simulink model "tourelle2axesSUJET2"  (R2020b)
settings: Solver=VariableStepAuto  StartTime=0.0  StopTime=0.2  RelTol=1e-3  AbsTol=1e-3
libraries: nesl_utility x7, fl_lib x6, ee_lib x3, batteryecm_lib x1, sdl_lib x1

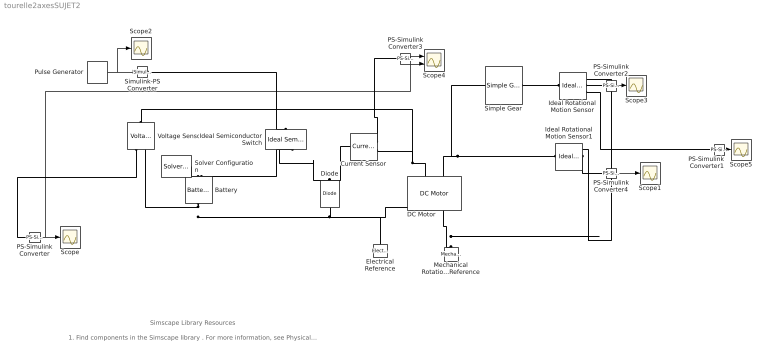
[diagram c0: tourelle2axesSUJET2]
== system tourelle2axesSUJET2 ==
  note: 1. Find components in the Simscape library . For more information, see Physical Modeling - Blocks . 2. Connect the components to form a physical network. For more information, see Essential Steps for Constructing a Physical Model . 3. Explore simulation results using sscexplore
  note: Simscape Library Resources
  Battery : batteryecm_lib/Battery  Vnom=3.93 V  prm_dir=simscape.enum.battery.prm_dir.disabled  R1_dis=2 Ohm  R1_ch=2 Ohm  R1=0.06 Ohm  prm_AH=2  AH=0.750 hr*A  V1=3.8 V  AH1=0.3 hr*A  prm_R2=simscape.enum.battery.prm_R2.enabled  R2=inf Ohm  Tmeas=298.15 K  charge_measurement_port=simscape.enum.battery.enable.no  prm_dyn=1  Rp1=0.005 Ohm  tau1=30 s  Rp2=0.005 Ohm  tau2=30 s  Rp3=0.005 Ohm  tau3=30 s  Rp4=0.005 Ohm  tau4=30 s  Rp5=0.005 Ohm  tau5=30 s  prm_fade=1  N_fade=100  AH_fade=45 hr*A  R1_fade=2.02 Ohm  R1_ch_fade=2.02 Ohm  V1_fade=10.35 V  prm_age=simscape.enum.battery.prm_age.disabled  prm_age_OCV=simscape.enum.battery.prm_age_OCV.OCV  OCV_age=0.9  SOC_age=60  Tmeas_age=298.15 K  delta_time_age_vec=[0] d  temperature_age_vec=[273] K  OCV_scaling_age=2.2134e6  OCV_offset_age=1.632e6  temp_exp_age=0.515833569 V  t_exp_age=0.75  Vnom_T2=12 V  R1_T2=2.2 Ohm  R1_T2_dis=2.2 Ohm  R1_T2_ch=2.2 Ohm  V1_T2=11.4 V  R2_T2=2200 Ohm  Rp1_T2=0.005 Ohm  tau1_T2=30 s  Rp2_T2=0.005 Ohm  tau2_T2=30 s  Rp3_T2=0.005 Ohm  tau3_T2=30 s  Rp4_T2=0.005 Ohm  tau4_T2=30 s  Rp5_T2=0.005 Ohm  tau5_T2=30 s  Tmeas2=273.15 K  thermal_port=simscape.enum.thermaleffects.omit  thermal_mass=30000 J/K  i_specify=off  i_priority=None  i=0 A  i_nominal_specify=off  i_nominal_value=1  i_nominal_unit=A  v_specify=off  v_priority=None  v=0 V  v_nominal_specify=off  v_nominal_value=1  v_nominal_unit=V  charge_specify=off  charge_priority=High  charge=50 hr*A  charge_nominal_specify=off  charge_nominal_value=1  charge_nominal_unit=hr*A  num_cycles_specify=off  num_cycles_priority=High  num_cycles=0  num_cycles_nominal_specify=off  num_cycles_nominal_value=1  num_cycles_nominal_unit=1  temperature_specify=off  temperature_priority=High  temperature=298.15 K  temperature_nominal_specify=off  temperature_nominal_value=1  temperature_nominal_unit=K
  Current Sensor : fl_lib/Electrical/Electrical Sensors/Current Sensor
  DC Motor : ee_lib/Electromechanical/Brushed Motors/DC Motor  field_option=ee.enum.field_option.pm  Rf=100 Ohm  Lf=1 H  Laf=0.15 H  If0=0 A  parameterization=1  Ra=79 Ohm  La=3 mH  emf_or_torque=1  Kv=0.0145 V/(rad/s)  Ki=6.876e-4 N*m/A  T_stall=0.24e-3 N*m  w_max=19100 rpm  w_rated=15000 rpm  P_rated=0.08 W  V_rated=1.5 V  lam_param=1  i_noload=0 A  V_i_noload=1.5 V  J=1 g*cm^2  lam=0 N*m/(rad/s)  speed0=0 rpm  enable_fault_armature=simscape.enum.onoff.off  rev_faulted=1 / 3  G_faulted_armature=1e-5 S  fault_trigger_armature=ee.enum.faults.faultTrigger.temporal  t_fault_armature=1 s  max_permissible_current_armature=inf A  t_fail_on_current_armature=1 s  enable_fault_field=simscape.enum.onoff.off  G_faulted_field=1e-5 S  fault_trigger_field=ee.enum.faults.faultTrigger.temporal  t_fault_field=1 s  max_permissible_current_field=inf A  t_fail_on_current_field=1 s  fault_action=simscape.enum.assert.action.none  alpha=3.93e-3 1/K  Tmeas=25 degC  thermal_mass=100 J/K  initial_temperature=25 degC
  Diode : ee_lib/Semiconductors & Converters/Diode  ModelType=ee.enum.diode.modelType.pwl  TableType=ee.enum.diode.tableType.IfMat  IfMat=[.07, .12, .19, 1.75, 4.24, 7.32, 11.2; .16, .3, .72, 2.14, 5.02, 8.35, 13.12] A  VfMat=[.9, 1.15, 1.25, 1.5, 1.75, 2.17, 2.6, 2.85; .58, .68, .75, 1.1, 1.38, 1.77, 2.27, 2.7] V  TjVec=[25, 125] degC  VfVec=[.5, .7, .9, 1.3, 1.7, 2.1, 2.5] V  IfVec=[.1, .2, .5, 1, 2, 4, 7, 10] A  IrMat=[1e-06, 2e-06, 5e-06, 1e-05, 2.5e-05, 5e-05, .0001; 2e-06, 5e-06, 1e-05, 4e-05, 8e-05, .0002, .0005] A  VrMat=[10, 100, 200, 250, 300, 325, 350; 10, 70, 160, 220, 270, 300, 320] V  VrVec=[10, 20, 40, 50, 70, 80, 100] V  IrVec=[1e-06, 2e-06, 5e-06, 1e-05, 2e-05, 5e-05, .0001] A  Vf=0.6 V  Ron=0.3 Ohm  Goff=1e-8 S  prmExp=ee.enum.diode.expParam.useTwo  I12=[.0137, .545] A  V12=[.6, .7] V  RS=0 Ohm  Tmeas=25 degC  IS=1e-12 A  ec=1  I1=0.0137 A  V1=0.6 V  N_series=1  N_parallel=1  ZenerEnable=false  Rz=0.3 Ohm  BV=inf V  C_param=ee.enum.diode.capParam.fixed  CJ=5 pF  CJ0=5 pF  Vvec=[.1, 10, 100] V  Cvec=[3.5, 1, .4] pF  VJ=1 V  Mgrad=0.5  FC=0.5  Q_param=ee.enum.diode.recoveryParam.off  iRM=-7.15 A  iF=4 A  didt=-750 A/us  trr_factor=3  trr=115 ns  Qrr=1500 s*uA  Vr=-600 V  Ls=150 nH  Erec=0.03 J  TT=50 ns  tau=100 ns  T_param=ee.enum.diode.temperatureParam.off  Tdevice=25 degC  I1_T2=0.245 A  V1_T2=0.5 V  IS_T2=1.25e-7 A  Tmeas2=125 degC  XTI_param=ee.enum.diode.xtiParam.pn  XTI=3  EG_param=ee.enum.diode.egapParam.material_si  EG=1.11 eV  dBVdT=0 V/K  enable_faults=simscape.enum.onoff.off  fault_action=simscape.enum.assert.action.none  fault_types=ee.enum.diode.faults.open  tau_fault=1e-3 s  IfMat_faulted=[.07, .12, .19, 1.75, 4.24, 7.32, 11.2; .16, .3, .72, 2.14, 4.02, 6.35, 9.12] A  VfMat_faulted=[.9, 1.15, 1.25, 1.5, 1.75, 2.17, 2.6, 2.85; .58, .68, .75, 1.1, 1.38, 1.77, 2.27, 2.7] V  VfVec_faulted=[.5, .7, .9, 1.3, 1.7, 2.1, 2.5] V  IfVec_faulted=[.1, .2, .5, 1, 2, 4, 7, 10] A  IrMat_faulted=[1e-06, 2e-06, 5e-06, 1e-05, 2.5e-05, 5e-05, .0001; 2e-06, 5e-06, 1e-05, 4e-05, 8e-05, .0002, .0005] A  VrMat_faulted=[1, 10, 20, 25, 30, 32.5, 35; 1, 5, 10, 20, 25, 30, 32] V  VrVec_faulted=[1, 2, 4, 5, 7, 8, 10] V  IrVec_faulted=[1e-06, 2e-06, 5e-06, 1e-05, 2e-05, 5e-05, .0001] A  Ropen_faulted=1000 Ohm  Gshort_faulted=1000 1/Ohm  Vf_faulted=0.6 V  Ron_faulted=0.3 Ohm  Goff_faulted=1e-8 S  I12_faulted=[.0137, .545] A  V12_faulted=[.6, .7] V  IS_faulted=1e-12 A  ec_faulted=1  I1_faulted=0.0137 A  V1_faulted=0.6 V  RS_faulted=0 Ohm  Rz_faulted=0.3 Ohm  BV_faulted=inf V  Cscale_faulted=100  fault_trigger=ee.enum.faults.faultTrigger.temporal  t_fault=inf s  max_permissible_voltage=inf V  n_fail_on_voltage=1  max_permissible_current=inf A  t_fail_on_current=1 s  max_permissible_dVdt=inf V/s  enable_fault_input=simscape.enum.onoff.off  i_specify=off  i_priority=None  i=0 A  i_nominal_specify=off  i_nominal_value=1  i_nominal_unit=A  v_specify=off  v_priority=None  v=0 V  v_nominal_specify=off  v_nominal_value=1  v_nominal_unit=V  v_capacitor_specify=off  v_capacitor_priority=None  v_capacitor=0 V  v_capacitor_nominal_specify=off  v_capacitor_nominal_value=1  v_capacitor_nominal_unit=V  Qj_specify=off  Qj_priority=High  Qj=0 C  Qj_nominal_specify=off  Qj_nominal_value=1  Qj_nominal_unit=C  faulted_specify=off  faulted_priority=None  faulted=0  faulted_nominal_specify=off  faulted_nominal_value=1  faulted_nominal_unit=1  i_diode_specify=off  i_diode_priority=None  i_diode=0 A  i_diode_nominal_specify=off  i_diode_nominal_value=1  i_diode_nominal_unit=A  v_diode_specify=off  v_diode_priority=None  v_diode=0 V  v_diode_nominal_specify=off  v_diode_nominal_value=1  v_diode_nominal_unit=V  i_capacitor_specify=off  i_capacitor_priority=None  i_capacitor=0 A  i_capacitor_nominal_specify=off  i_capacitor_nominal_value=1  i_capacitor_nominal_unit=A  power_dissipated_specify=off  power_dissipated_priority=None  power_dissipated=0 W  power_dissipated_nominal_specify=off  power_dissipated_nominal_value=1  power_dissipated_nominal_unit=W  fidelity_level=ee.enum.diode.fidelity.includeChargeDyn  rec_loss_model=ee.enum.diode.reverseRecoveryModel.fixed  ErecVal=0 J  scaleWithIandV=true  ErecMat=zeros(2, 3) J  TjrecVec=[298.15, 398.15] K  IfrecVec=[.1, 1, 10] A  IrecVal=10 A  VrecVal=10 V  tFilter=1 / 1000 / 100 s  max_permissible_temperature=inf K  t_fail_on_temperature=1 s  thermal_network_parameterization=ee.enum.thermalNetworkTopology.cauer  Rth=[0, 10] K/W  Rth_Cauer=[1, 3, 10] K/W  Rth_Foster=[4, 6] K/W  thermal_mass_parameterization=ee.enum.thermalNetwork.timeconstant  thermal_mass=[0, 1] J/K  thermal_mass_Cauer=[.1, .3, 1] J/K  thermal_mass_Foster=[1.5, 3] J/K  thermal_time_constant=[0, 10] s  thermal_time_constant_Cauer=[1, 3, 10] s  thermal_time_constant_Foster=[6, 18] s  thermal_mass_initial_temperatures=[25, 25] degC  thermal_mass_initial_temperatures_Cauer=[25, 25, 25] degC  junction_thermal_mass=0.01 J/K  Tvec_initial_Foster=[25, 25, 25, 25] degC  no_thermal_network=0  junction_temperature_specify=off  junction_temperature_priority=None  junction_temperature=25 degC  junction_temperature_nominal_specify=off  junction_temperature_nominal_value=1  junction_temperature_nominal_unit=degC
  Electrical Reference : fl_lib/Electrical/Electrical Elements/Electrical Reference
  Ideal Rotational Motion Sensor : fl_lib/Mechanical/Mechanical Sensors/Ideal Rotational Motion Sensor  reference=foundation.enum.MeasurementReference.difference  acceleration_port=false  velocity_port=true  position_port=true  wrap_angle=false  offset=0 rad
  Ideal Rotational Motion Sensor1 : fl_lib/Mechanical/Mechanical Sensors/Ideal Rotational Motion Sensor  reference=foundation.enum.MeasurementReference.difference  acceleration_port=false  velocity_port=true  position_port=true  wrap_angle=false  offset=0 rad
  Ideal Semiconductor Switch : ee_lib/Semiconductors & Converters/Ideal Semiconductor Switch  port_option=ee.enum.controlport.ps  Ron=0.001 Ohm  Goff=1e-6 1/Ohm  Vth=0.5 V  diode_param=1  diode_Vf=0.8 V  diode_Ron=0.001 Ohm  diode_Goff=1e-5 1/Ohm  diode_C=50e-9 F  diode_iRM=-235 A  diode_iF=300 A  diode_idot=-50 A/us  diode_trr_param=1  diode_trr_factor=3  diode_trr=15 us  diode_Qrr=1500 s*uA
  Mechanical Rotational Reference : fl_lib/Mechanical/Rotational Elements/Mechanical Rotational Reference
  PS-Simulink Converter : nesl_utility/PS-Simulink Converter  PhysicalDomain=network_engine_domain  SubClassName=ps_output  LeftPortType=input  RightPortType=output  PseudoPeriodic=off  Frequencies=[]  VectorFormat=1-D array  Unit=V  AffineConversion=off
  PS-Simulink Converter1 : nesl_utility/PS-Simulink Converter  PhysicalDomain=network_engine_domain  SubClassName=ps_output  LeftPortType=input  RightPortType=output  PseudoPeriodic=off  Frequencies=[]  VectorFormat=1-D array  Unit=inherit  AffineConversion=off
  PS-Simulink Converter2 : nesl_utility/PS-Simulink Converter  PhysicalDomain=network_engine_domain  SubClassName=ps_output  LeftPortType=input  RightPortType=output  PseudoPeriodic=off  Frequencies=[]  VectorFormat=1-D array  Unit=rad/s  AffineConversion=off
  PS-Simulink Converter3 : nesl_utility/PS-Simulink Converter  PhysicalDomain=network_engine_domain  SubClassName=ps_output  LeftPortType=input  RightPortType=output  PseudoPeriodic=off  Frequencies=[]  VectorFormat=1-D array  Unit=inherit  AffineConversion=off
  PS-Simulink Converter4 : nesl_utility/PS-Simulink Converter  PhysicalDomain=network_engine_domain  SubClassName=ps_output  LeftPortType=input  RightPortType=output  PseudoPeriodic=off  Frequencies=[]  VectorFormat=1-D array  Unit=rad/s  AffineConversion=off
  Pulse Generator : DiscretePulseGenerator  PulseType=Time based  Amplitude=6  Period=5e-3  PulseWidth=75
  Scope{,1..3,5} (5 alike) : Scope
  Scope4 : Scope  NumInputPorts=2
  Simple Gear : sdl_lib/Gears/Simple Gear  ratio=516.6  rotation_direction=3-2*(1)  enable_faults=simscape.enum.onoff.off  efficiency_fault=0.05  fault_angles=pi / 12 rad  friction_model=sdl.enum.gear_efficiencies_load.off  T_noload=0.1 N*m  T_nom=5 N*m  efficiency_nom=0.8  efficiency=0.8  temperature_TLU=[280, 300, 320] K  load_TLU=[1, 5, 10] N*m  efficiency_TLU=[.95, .9, .85]  efficiency_TLU2=[.85, .8, .75; .95, .9, .85; .85, .8, .7]  w_thr=0.01 rad/s  pwr_thr=0.001 W  enable_backlash=false  hardstop_model=simscape.enum.hardstop.smooth  backlash_distance=1e-3 mm  r_base=0.1 m  transition=1e-4 mm  backlash_stiffness=1e6 N/m  backlash_damping=1e3 N*s/m  coeff_rest=0.7  v_tol=0.001 m/s  f_tol=0 N  mu_visc=[0.000000763, 0] N*m/(rad/s)  thermal_mass=50 J/K  temperature_specify=off  temperature_priority=High  temperature=300 K  temperature_nominal_specify=off  temperature_nominal_value=1  temperature_nominal_unit=K  x_backlash_specify=off  x_backlash_priority=None  x_backlash=0 mm  x_backlash_nominal_specify=off  x_backlash_nominal_value=1  x_backlash_nominal_unit=mm  f_hardstop_specify=off  f_hardstop_priority=None  f_hardstop=0 N  f_hardstop_nominal_specify=off  f_hardstop_nominal_value=1  f_hardstop_nominal_unit=N  v_backlash_specify=off  v_backlash_priority=None  v_backlash=0 m/s  v_backlash_nominal_specify=off  v_backlash_nominal_value=1  v_backlash_nominal_unit=m/s
  Simulink-PS Converter : nesl_utility/Simulink-PS Converter  PhysicalDomain=network_engine_domain  SubClassName=ps_input  LeftPortType=input  RightPortType=output  PseudoPeriodic=off  Frequencies=[]  NoiseDistribution=none  NoiseParameters=[]  Unit=1  AffineConversion=off  FilteringAndDerivatives=provide  SimscapeFilterOrder=1  InputFilterTimeConstant=0.001  UdotUserProvided=0
  Solver Configuration : nesl_utility/Solver Configuration  PhysicalDomain=network_engine_domain  SubClassName=solver  LeftPortType=input  RightPortType=generic  Tones=[]  Harmonics=[]  SimulateNoise=off  Profile=off  UseLocalSampling=off  EnableSwitchedLinearOptims=on  FrequencyDomain=off  UseCCode=off  RelTol=0.001  AbsTol=1e-06  MinStep=1e-09  ToWorkspace=off  RevertToSquareIcSolve=off  NumHomotopyIterations=100  PhasorMode=off  PhasorModeNumHarmonics=1  ConsistencySolver=NEWTON_FTOL  IndexReductionMethod=DerivativeReplacement  DoDC=off  ResidualTolerance=1e-09  ConsistencyTolSource=GLOBAL  ConsistencyAbsTol=0.001  ConsistencyRelTol=0.001  ConsistencyTolFactor=0.001  UseLocalSolver=off  LocalSolverChoice=NE_BACKWARD_EULER_ADVANCER  ResolveIndetEquations=on  FunctionEvalNumThread=1  LocalSolverSampleTime=0.001  DoFixedCost=off  MaxNonlinIter=3  MaxModeIter=2  ComputeImpulses=off  ImpulseIterations=2  LinearAlgebra=auto  LinearAlgebraNumThread=0  EquationFormulation=NE_TIME_EF  DelaysMemoryBudget=1024  AutomaticFiltering=on  FilteringTimeConstant=0.001  PartitionStorageMethod=AS_NEEDED  PartitionMemoryBudget=1024  PartitionMethod=ROBUST  MultibodyUseLocalSolver=off  MultibodyLocalSolverChoice=ODE1  MultibodyLocalSolverSampleTime=0.001
  Voltage Sensor : fl_lib/Electrical/Electrical Sensors/Voltage Sensor
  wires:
  PS-Simulink Converter/1 -> Scope4/2, Scope/1
  Pulse Generator/1 -> Scope2/1, Simulink-PS Converter/1
  PS-Simulink Converter2/1 -> Scope3/1
  PS-Simulink Converter3/1 -> Scope4/1
  PS-Simulink Converter4/1 -> Scope1/1
  PS-Simulink Converter1/1 -> Scope5/1
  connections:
  Battery/RConn1 -- DC Motor/RConn1 -- Electrical Reference/LConn1 -- Diode/LConn1 -- Voltage Sensor/RConn2
  Diode/RConn1 -- Current Sensor/LConn1 -- Ideal Semiconductor Switch/RConn1
  Voltage Sensor/RConn1 -- PS-Simulink Converter/LConn1
  Ideal Rotational Motion Sensor/RConn2 -- PS-Simulink Converter2/LConn1
  Voltage Sensor/LConn1 -- DC Motor/LConn1 -- Current Sensor/RConn2
  Current Sensor/RConn1 -- PS-Simulink Converter3/LConn1
  Mechanical Rotational Reference/LConn1 -- DC Motor/RConn2 -- Ideal Rotational Motion Sensor1/RConn1 -- Ideal Rotational Motion Sensor/RConn1
  Ideal Rotational Motion Sensor1/LConn1 -- DC Motor/LConn2 -- Simple Gear/LConn1
  Ideal Rotational Motion Sensor1/RConn2 -- PS-Simulink Converter4/LConn1
  Simple Gear/RConn1 -- Ideal Rotational Motion Sensor/LConn1
  Ideal Rotational Motion Sensor/RConn3 -- PS-Simulink Converter1/LConn1
  Simulink-PS Converter/RConn1 -- Ideal Semiconductor Switch/LConn1
  Battery/LConn1 -- Solver Configuration/RConn1 -- Ideal Semiconductor Switch/RConn2
